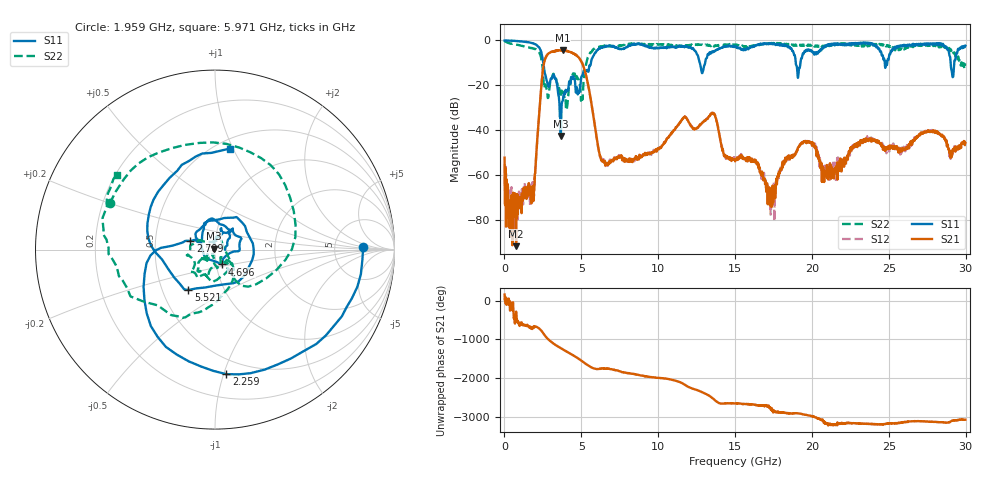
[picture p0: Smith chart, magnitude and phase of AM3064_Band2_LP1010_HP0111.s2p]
# Hz S DB R 50.0
!freq dBS11 angS11 dBS21 angS21 dBS12 angS12 dBS22 angS22
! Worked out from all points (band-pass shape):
!   1600 points, 10 MHz to 29.98 GHz, reference 50 ohm
!   highest |S21| = -4.36 dB at 3.777 GHz (marker M1); lowest = -91.5 dB at 759.8 MHz (marker M2)
!   |S21| within 3 dB of the highest: 2.7 GHz to 4.8 GHz (2.099 GHz wide, 56 % of centre)
!   lowest |S11| = -42.6 dB at 3.665 GHz (marker M3), VSWR 1.02, Z = 49.4 + j0.44 ohm
!   |S11| at or under -10 dB: 2.53 GHz to 5.623 GHz (3.093 GHz wide, 75.9 % of centre); 12.7 GHz to 13.06 GHz (350.3 MHz wide, 2.72 % of centre); 18.95 GHz to 19.25 GHz (304.1 MHz wide, 1.59 % of centre)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
!   |S22| runs from -30.7 to -0.3 dB; largest |S21 - S12| = 0.021
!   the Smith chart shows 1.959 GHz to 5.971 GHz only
!   S11 on the Smith chart (normalised r, x): 1.959 GHz: 10, +1; 2.259 GHz: 0.38, -1.02; 2.709 GHz: 0.76, +0.07; 4.696 GHz: 1.07, -0.18; 5.521 GHz: 0.68, -0.33; 5.971 GHz: 0.58, +0.97
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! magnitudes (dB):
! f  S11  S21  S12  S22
! 10 MHz  -0.1  -52.1  -55.3  -0.3
! 759.8 MHz  -0.3  -91.5  -69.2  -1.9
! 1.959 GHz  -1.7  -64.6  -62.0  -3.9
! 2.259 GHz  -3.1  -32.6  -32.5  -5.2
! 2.709 GHz  -16.8  -7.3  -7.2  -20.6
! 3.665 GHz  -42.6  -4.4  -4.4  -24.1
! 3.777 GHz  -27.0  -4.4  -4.5  -24.5
! 4.696 GHz  -20.8  -6.8  -6.8  -15.9
! 5.015 GHz  -16.0  -9.6  -9.5  -24.8
! 5.521 GHz  -11.4  -22.7  -22.6  -6.4
! 5.971 GHz  -4.9  -42.0  -42.4  -3.3
! 6.627 GHz  -2.6  -55.1  -54.5  -2.5
! 10 GHz  -3.4  -48.3  -48.3  -1.8
! 13.54 GHz  -5.4  -32.3  -32.2  -2.6
! 15 GHz  -2.7  -53.8  -52.9  -1.8
! 17.4 GHz  -1.6  -73.6  -71.7  -1.4
! 19.99 GHz  -4.7  -46.3  -45.9  -1.9
! 20.8 GHz  -2.6  -63.0  -61.0  -2.5
! 25 GHz  -8.0  -47.5  -47.4  -2.2
! 28.39 GHz  -1.3  -42.0  -42.3  -3.0
! 29.18 GHz  -16.3  -49.1  -49.6  -4.7
! 29.98 GHz  -2.4  -45.6  -45.3  -10.2
